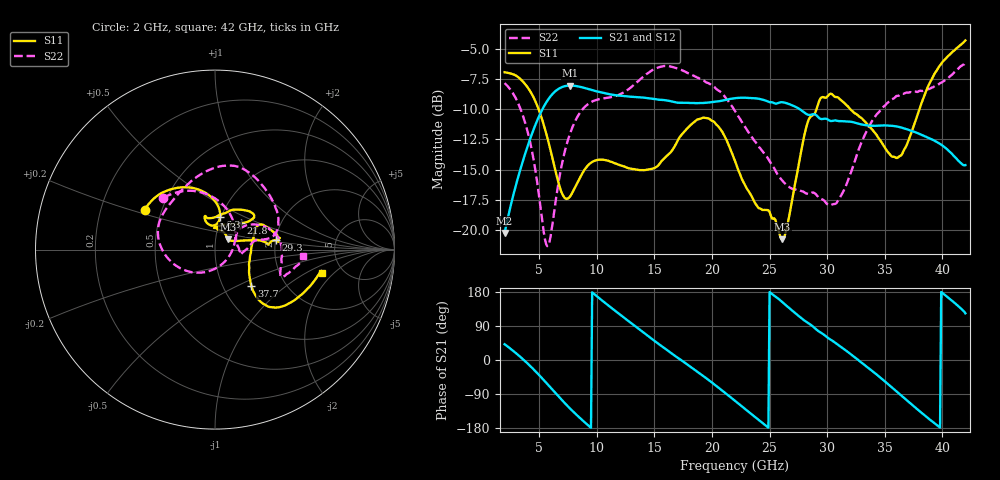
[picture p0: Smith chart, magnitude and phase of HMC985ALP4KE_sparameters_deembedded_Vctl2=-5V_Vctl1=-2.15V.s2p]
!s2p File: Measurements: S11, S21, S12, S22
# GHz S dB R 50.0
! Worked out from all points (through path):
!   401 points, 2 GHz to 42 GHz, reference 50 ohm
!   highest |S21| = -8.02 dB at 7.7 GHz (marker M1); lowest = -20.3 dB at 2 GHz (marker M2)
!   lowest |S11| = -20.8 dB at 26.1 GHz (marker M3), VSWR 1.20, Z = 57.3 + j6.56 ohm
!   |S11| at or under -10 dB: 4.957 GHz to 29.07 GHz (24.11 GHz wide, 142 % of centre); 32.02 GHz to 38 GHz (5.978 GHz wide, 17.1 % of centre)
!   |S22| runs from -21.4 to -6.1 dB; largest |S21 - S12| = 0.00051
!   S11 on the Smith chart (normalised r, x): 2 GHz: 0.40, +0.22; 6.3 GHz: 0.99, +0.37; 21.8 GHz: 1.27, +0.39; 29.3 GHz: 2.00, +0.24; 37.7 GHz: 1.36, -0.60; 42 GHz: 3.50, -1.46
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2  -6.91 150.5  -20.28 41.7  -20.28 41.7  -7.81 134.9
3.3  -7.42 129.9  -15.21 9.9  -15.21 10.0  -9.78 102.4
4.6  -9.18 105.5  -11.46 -27.3  -11.46 -27.3  -14.63 56.2
5.6  -11.96 87.3  -9.45 -59.8  -9.45 -59.8  -21.18 -23.9
6.3  -14.65 81.2  -8.58 -83.4  -8.59 -83.4  -18.52 -101.1
7.7  -17.21 100.5  -8.02 -128.6  -8.02 -128.6  -11.95 -164.2
8.7  -15.39 108.3  -8.16 -157.5  -8.16 -157.5  -10.07 172.3
12.2  -14.69 104.6  -8.88 115.6  -8.89 115.6  -8.66 125.2
15.4  -14.58 86.2  -9.20 41.7  -9.20 41.8  -6.50 81.6
18.4  -11.09 51.3  -9.48 -23.7  -9.48 -23.6  -7.21 49.0
21.8  -13.78 45.7  -9.09 -102.8  -9.10 -102.7  -9.83 12.5
22  -14.28 48.4  -9.07 -107.7  -9.07 -107.7  -10.13 11.9
24.1  -18.22 89.1  -9.12 -159.1  -9.13 -159.1  -13.14 11.9
26.1  -20.81 38.5  -9.40 153.0  -9.41 153.0  -15.91 -3.8
28.7  -10.51 5.2  -10.41 90.0  -10.42 90.0  -16.91 -6.6
29.3  -9.32 8.8  -10.72 75.0  -10.72 75.0  -17.36 -2.1
30.8  -8.98 12.7  -10.94 43.0  -10.94 43.1  -17.80 24.8
32.4  -10.33 26.1  -11.10 7.0  -11.10 7.1  -14.30 39.5
35.4  -13.68 6.8  -11.35 -66.6  -11.35 -66.5  -9.35 16.2
37.7  -10.88 -44.9  -11.91 -126.7  -11.91 -126.6  -8.52 -6.4
39.8  -6.33 -41.7  -12.87 -178.3  -12.87 -178.2  -7.82 -21.9
42  -4.27 -12.3  -14.63 123.0  -14.63 123.1  -6.12 -4.3
